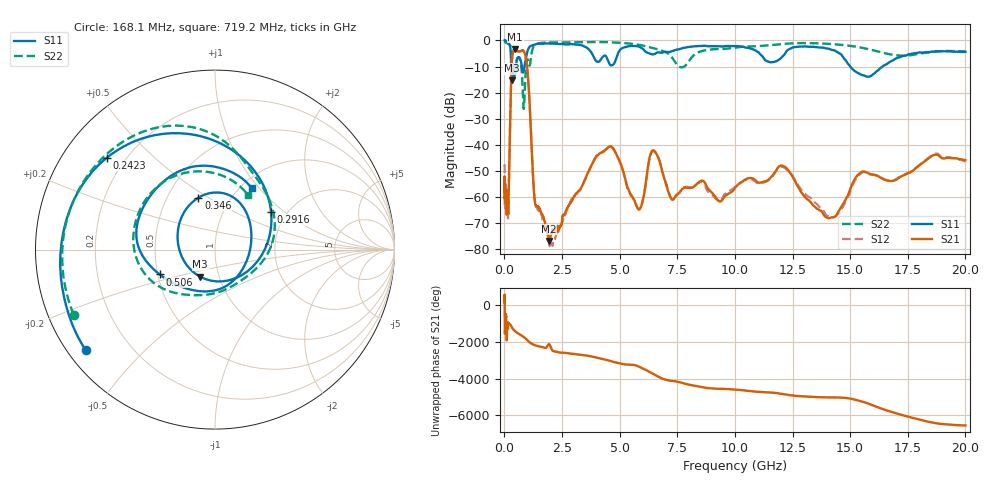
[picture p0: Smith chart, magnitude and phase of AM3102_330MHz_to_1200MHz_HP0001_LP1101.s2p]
! Date/Time: Tue, Sep 11, 2018 5:10 PM
! Network Analyzer: Agilent Technologies E8362B Rev: A.07.50.63
! Sweep from 0.010 to 20.000 GHz, 1601 Points, Sweep Type: LOG
! Power Supply: 4.950 V, 0.001 A
# Hz S DB R 50
!freq MagS11 AngS11 MagS21 AngS21 MagS12 AngS12 MagS22 AngS22
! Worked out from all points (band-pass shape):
!   1601 points, 10 MHz to 20 GHz, reference 50 ohm
!   highest |S21| = -3.21 dB at 464.5 MHz (marker M1); lowest = -76.7 dB at 1.932 GHz (marker M2)
!   |S21| within 3 dB of the highest: 336.6 MHz to 922.1 MHz (585.5 MHz wide, 93 % of centre)
!   lowest |S11| = -15.3 dB at 316.2 MHz (marker M3), VSWR 1.42, Z = 40.6 - j12.7 ohm
!   |S11| at or under -10 dB: 360.8 MHz to 499 MHz (138.2 MHz wide, 32.2 % of centre); 759.1 MHz to 869.9 MHz (110.8 MHz wide, 13.6 % of centre); 15.01 GHz to 16.4 GHz (1.393 GHz wide, 8.87 % of centre)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
!   |S22| runs from -26.2 to -0.3 dB; largest |S21 - S12| = 0.012
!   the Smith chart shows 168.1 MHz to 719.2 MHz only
!   S11 on the Smith chart (normalised r, x): 168.1 MHz: 0.05, -0.34; 242.3 MHz: 0.13, +0.36; 291.6 MHz: 1.66, +0.81; 346 MHz: 0.71, +0.45; 506 MHz: 0.51, -0.16; 719.2 MHz: 1.12, +0.91
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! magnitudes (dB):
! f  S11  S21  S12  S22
! 10 MHz  0.0  -53.5  -47.9  -0.3
! 35.55 MHz  0.0  -61.9  -59.7  -0.6
! 126.4 MHz  -0.4  -63.1  -64.4  -1.1
! 168.1 MHz  -0.8  -65.3  -65.4  -1.2
! 242.3 MHz  -2.0  -34.8  -35.0  -1.8
! 291.6 MHz  -8.5  -14.3  -14.4  -3.4
! 316.2 MHz  -15.3  -8.3  -8.3  -5.5
! 346 MHz  -10.3  -5.7  -5.7  -7.6
! 447.2 MHz  -13.3  -3.2  -3.3  -12.4
! 464.5 MHz  -12.4  -3.2  -3.2  -11.6
! 506 MHz  -9.4  -3.4  -3.5  -9.2
! 719.2 MHz  -8.0  -4.0  -4.0  -9.0
! 837.2 MHz  -11.7  -4.1  -4.1  -26.2
! 984 MHz  -4.7  -10.1  -10.1  -7.6
! 1.309 GHz  -1.5  -60.5  -60.4  -1.8
! 1.59 GHz  -1.3  -66.0  -66.1  -0.9
! 1.932 GHz  -1.2  -76.7  -77.0  -0.8
! 4.5 GHz  -7.7  -41.0  -40.8  -0.6
! 5.652 GHz  -2.1  -61.4  -61.1  -1.4
! 6.518 GHz  -5.2  -42.3  -42.6  -3.1
! 14.07 GHz  -3.2  -68.0  -67.3  -1.3
! 20 GHz  -4.4  -45.8  -46.4  -4.2
